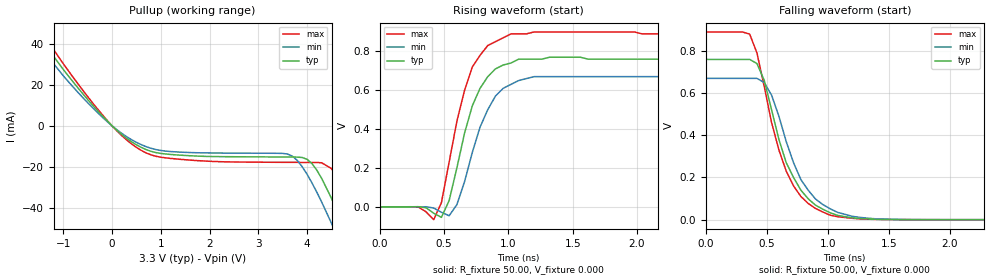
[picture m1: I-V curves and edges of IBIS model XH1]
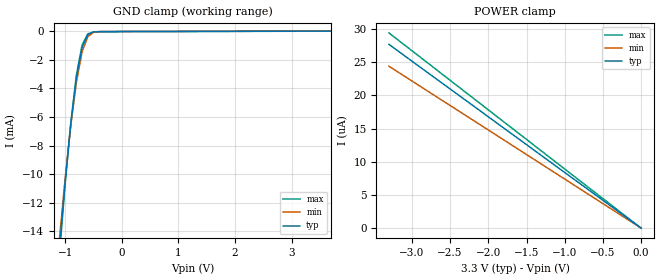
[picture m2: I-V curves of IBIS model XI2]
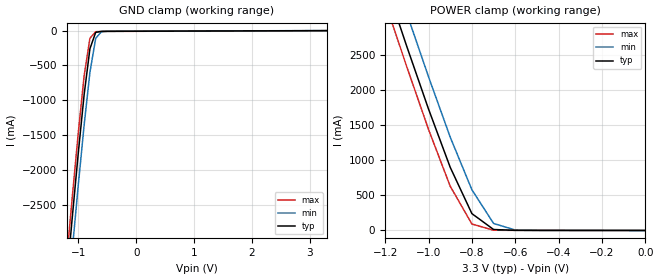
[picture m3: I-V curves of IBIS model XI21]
|   * 9db801b.ibs * IBIS 2.1 Model file
| Rev History
| Rev No.   Description
| 1.0   Initial release
| 1.1   Updated Parasitic Parameters,
|   Input and output C_comp min / Max tightened + Added pin RLC
[IBIS Ver]   2.1
[Comment char]  |_char
[File name]   9db801b.ibs
[Date]   November,2 2004
[File Rev]   1.0
[Source]   Originated at Integrated Circuit Systems, Inc.
[Disclaimer] (C) Copyright Integrated Circuit Systems, Inc. 2004
   All rights reserved
ICS hereby grants the user of this IBIS model a non-exclusive,
nontransferable license to use this IBIS model under the following terms.
Before using this IBIS model, the user should read this license.
If the user does not accept these terms,  the IBIS model should be
returned to ICS within 30 days.
   The user is granted this license only to use the IBIS model and
is not granted rights to sell, load, rent, lease or license the IBIS
model in whole or in part, or in modified form to anyone other than
user. User may modify the IBIS model to suit its specific
applications but rights to derivative works and such modifications
shall belong to ICS.
   This IBIS model is provided on an "AS IS" basis and ICS makes
absolutely no warranty with respect to the information contained
herein. ICS DISCLAIMS AND CUSTOMER WAIVES ALL WARRANTIES, EXPRESS
OR IMPLIED, INCLUDING WARRANTIES OF MERCHANTABILITY OR FITNESS FOR
A PARTICULAR PURPOSE. The entire risk as to quality and performance
is with the Customer. ACCORDINGLY, IN NO EVENT SHALL THE COMPANY BE
LIABLE FOR ANY DAMAGES, WHETHER IN CONTRACT OR TORT,INCLUDING ANY
LOST PROFITS OR OTHER INCIDENTAL, CONSEQUENTIAL, EXEMPLARY, OR
PUNITIVE DAMAGES ARISING OUT OF THE USE OR APPLICATION OF THE IBIS
model provided in this package. Further, ICS reserves the right to
make changes without notice to any product herein to improve
reliability, function, or design. ICS does not convey any license
under patent rights or any other intellectual property rights,
including those of third parties.
   ICS is not obligated to provide maintenance or support
for the licensed IBIS model.
|   COMPONENT: ICS9db801b
[Component]   ICS9db801b
[Manufacturer]  ICS
[Package]
| variable   typ   min   max
R_pkg   70.0m   50.0m   90.0m
L_pkg   5.1nH   3.2nH   7.0nH
C_pkg   0.70pF  0.50pF  0.90pF
[Pin]   signal_name   model_name   R_pin   L_pin   C_pin
  1   SRCDIVB   XI23
  2   VDD   POWER
  3   VSS   GND
  4   SRC_IN   XI4
  5   SRC_IN#   XI4
  6   OE_0(OE_0#)   XI21
  7   OE_3(OE_3#)   XI21
  8   DIF_0   XH1
  9   DIF_0#   XH1
 10   GND   GND
 11   VDD   POWER
 12   DIF_1   XH1
 13   DIF_1#   XH1
 14   OE_1(OE_1#)   XI23
 15   OE_2(OE_2#)   XI23
 16   DIF_2   XH1
 17   DIF_2#   XH1
 18   GND   GND
 19   VDD   POWER
 20   DIF_3   XH1
 21   DIF_3#   XH1
 22   BYPASS#/PLL   XI23
 23   SCLK   XI10
 24   SDATA   XIO3
 25   GND   GND
 26   PD#(PD)   XI2
 27   SRC_STOP#(SRC_STOP)   XI23
 28   HIGH_BW#   XI23
 29   DIF_4#   XH1
 30   DIF_4   XH1
 31   VDD   POWER
 32   GND   GND
 33   DIF_5#   XH1
 34   DIF_5   XH1
 35   OE_5(OE_5#)   XI23
 36   OE_6(OE_6#)   XI23
 37   DIF_6#   XH1
 38   DIF_6   XH1
 39   VDD   POWER
 40   OE_INV#(OE_INV)   XI24
 41   DIF_7#   XH1
 42   DIF_7   XH1
 43   OE_4(OE_4#)   XI21
 44   OE_7(OE_7#)   XI21
 45   LOCKOUT   XO1
 46   IREF   XI29
 47   GNDA   GND
 48   VDDA   POWER
|* Either 3.3V or 2.5V
|** All model are simulated with typical corner process
[Diff Pin]   inv_pin   vdiff   tdelay_typ
4   5   NA   NA
8   9   NA   NA
12   13   NA   NA
16   17   NA   NA
20   21   NA   NA
30   29   NA   NA
34   33   NA   NA
38   37   NA   NA
42   41   NA   NA
| Models and submodels in the file (10): XH1 (Open_source), XI2 (Input), XI21 (Input), XI23 (Input), XI24 (Input), XI29 (Input), XI10 (Input), XI4 (Input), XIO3 (I/O_open_drain), XO1 (Output)
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|   Model XH1
[Model]   XH1
Model_type   Open_source
Polarity   Inverting
C_comp   3.40pF   2.85pF   3.95pF
[Temperature Range]   25.00   70.00   0.000
[Voltage Range]   3.30V   3.00V   3.70V
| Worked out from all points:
|   slope of the pullup table from 0 to 0.495 V, typ, clamps not added: 53.7 ohm
|   rising waveform, R_fixture 50.00, V_fixture 0.000: 20-80 % time 196ps typ, 209ps min, 191ps max; typ from 0 V to 0.76 V
|   falling waveform, R_fixture 50.00, V_fixture 0.000: 20-80 % time 266ps typ, 276ps min, 255ps max; typ from 0.76 V to 0 V
[Pullup]
| voltage   I(typ)   I(min)   I(max)
-3.3V     120mA      110mA      120mA
-1.9V     57.97mA    52.49mA    62.98mA
-1.5V     43.73mA    39.31mA    47.78mA
-100mV    2.37mA     2.07mA     2.66mA
700mV     -11.65mA   -10.21mA   -13.27mA
3.6V      -15.27mA   -13.83mA   -17.88mA
4V        -16.4mA    -23.77mA   -17.93mA
4.3V      -25.83mA   -37.4mA    -18.11mA
4.5V      -35.53mA   -47.74mA   -20.97mA
4.7V      -46.5mA    -58.63mA   -28.65mA
5.1V      -70.24mA   -81.19mA   -50.61mA
6.6V      -160mA     -170mA     -150mA
[Ramp]
| variable   typ   min   max
dV/dt_r   0.46/0.20n   0.40/0.21n   0.53/0.19n
dV/dt_f   0.45/0.26n   0.40/0.27n   0.53/0.25n
R_load = 50.00
[Rising Waveform]
R_fixture = 50.00
V_fixture = 0.000
V_fixture_min = 0.000
V_fixture_max = 0.000
| time   V(typ)   V(min)   V(max)
0s        -370nV     -380nV     -340nV
300ps     550uV      230uV      -1.44mV
420ps     -32.86mV   -6.35mV    -66.34mV
480ps     -54.44mV   -28.27mV   21.55mV
540ps     32.24mV    -46.01mV   230mV
600ps     200mV      10.91mV    440mV
720ps     520mV      280mV      720mV
840ps     670mV      500mV      830mV
1.02ns    740mV      630mV      890mV
3ns       760mV      670mV      890mV
[Falling Waveform]
R_fixture = 50.00
V_fixture = 0.000
V_fixture_min = 0.000
V_fixture_max = 0.000
| time   V(typ)   V(min)   V(max)
0s        760mV      670mV      890mV
360ps     760mV      670mV      880mV
420ps     740mV      670mV      790mV
480ps     660mV      650mV      630mV
540ps     520mV      590mV      460mV
660ps     270mV      370mV      230mV
780ps     140mV      190mV      110mV
900ps     68.75mV    97.98mV    52.94mV
1.38ns    2.27mV     4.59mV     1.49mV
3ns       -13.74uV   -37.6uV    -15.05uV
|   Model XI2
[Model]   XI2
Model_type   Input
Polarity   Inverting
Vinl =   0.80V
Vinh =   2.00V
C_comp   3.40pF   2.85pF   3.95pF
[Temperature Range]   25.00   70.00   0.000
[Voltage Range]   3.30V   3.00V   3.70V
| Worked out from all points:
|   GND clamp passes 1 mA (typ) near -0.69 V on its own axis
[GND_clamp]
| voltage   I(typ)   I(min)   I(max)
-3.3V     -150mA     -140mA     -150mA
-1.1V     -15.17mA   -14.5mA    -15.62mA
-1V       -10.54mA   -10.3mA    -10.7mA
-900mV    -6.48mA    -6.58mA    -6.4mA
-800mV    -3.23mA    -3.54mA    -3.03mA
-700mV    -1.13mA    -1.43mA    -950uA
-600mV    -250uA     -390uA     -190uA
-500mV    -58.48uA   -85.04uA   -52.74uA
-400mV    -33.35uA   -32.48uA   -37.57uA
3.7V      170pA      5.18uA     140pA
[POWER_clamp]
| voltage   I(typ)   I(min)   I(max)
-3.3V     27.7uA     24.41uA    29.43uA
-3.2V     26.86uA    23.67uA    28.53uA
-2.7V     22.66uA    19.97uA    24.08uA
0V        140pA      2.62nA     140pA
|   Model XI21
[Model]   XI21
Model_type   Input
Polarity   Inverting
Enable   Active-High
Vinl =   0.80V
Vinh =   2.00V
C_comp   3.40pF   2.85pF   3.95pF
[Temperature Range]   27.00   70.00   0.000
[Voltage Range]   3.30V   3.00V   3.70V
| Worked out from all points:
|   POWER clamp passes 1 mA (typ) near -0.39 V on its own axis
[GND_clamp]
| voltage   I(typ)   I(min)   I(max)
-3.3V     -24.07A    -24.5A     -23.8A
-1.2V     -3.56A     -4.03A     -3.27A
-1.1V     -2.64A     -3.11A     -2.35A
-1V       -1.75A     -2.21A     -1.46A
-900mV    -920mA     -1.36A     -650mA
-800mV    -260mA     -600mA     -110mA
-700mV    -25mA      -110mA     -15.24mA
-600mV    -10.97mA   -15.13mA   -11.57mA
-500mV    -9.91mA    -9.4mA     -10.9mA
3.3V      450nA      780uA      -1.03mA
[POWER_clamp]
| voltage   I(typ)   I(min)   I(max)
-3.3V     24.04A     24.47A     23.78A
-1.2V     3.54A      4.01A      3.25A
-1.1V     2.62A      3.09A      2.33A
-1V       1.73A      2.19A      1.44A
-900mV    900mA      1.33A      630mA
-800mV    240mA      580mA      92.42mA
-700mV    13.81mA    100mA      3.74mA
-600mV    1.83mA     6.31mA     1.58mA
0V        130pA      310pA      130pA
